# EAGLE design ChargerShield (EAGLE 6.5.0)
Dings

## Sheet 1 of 2: User Interface
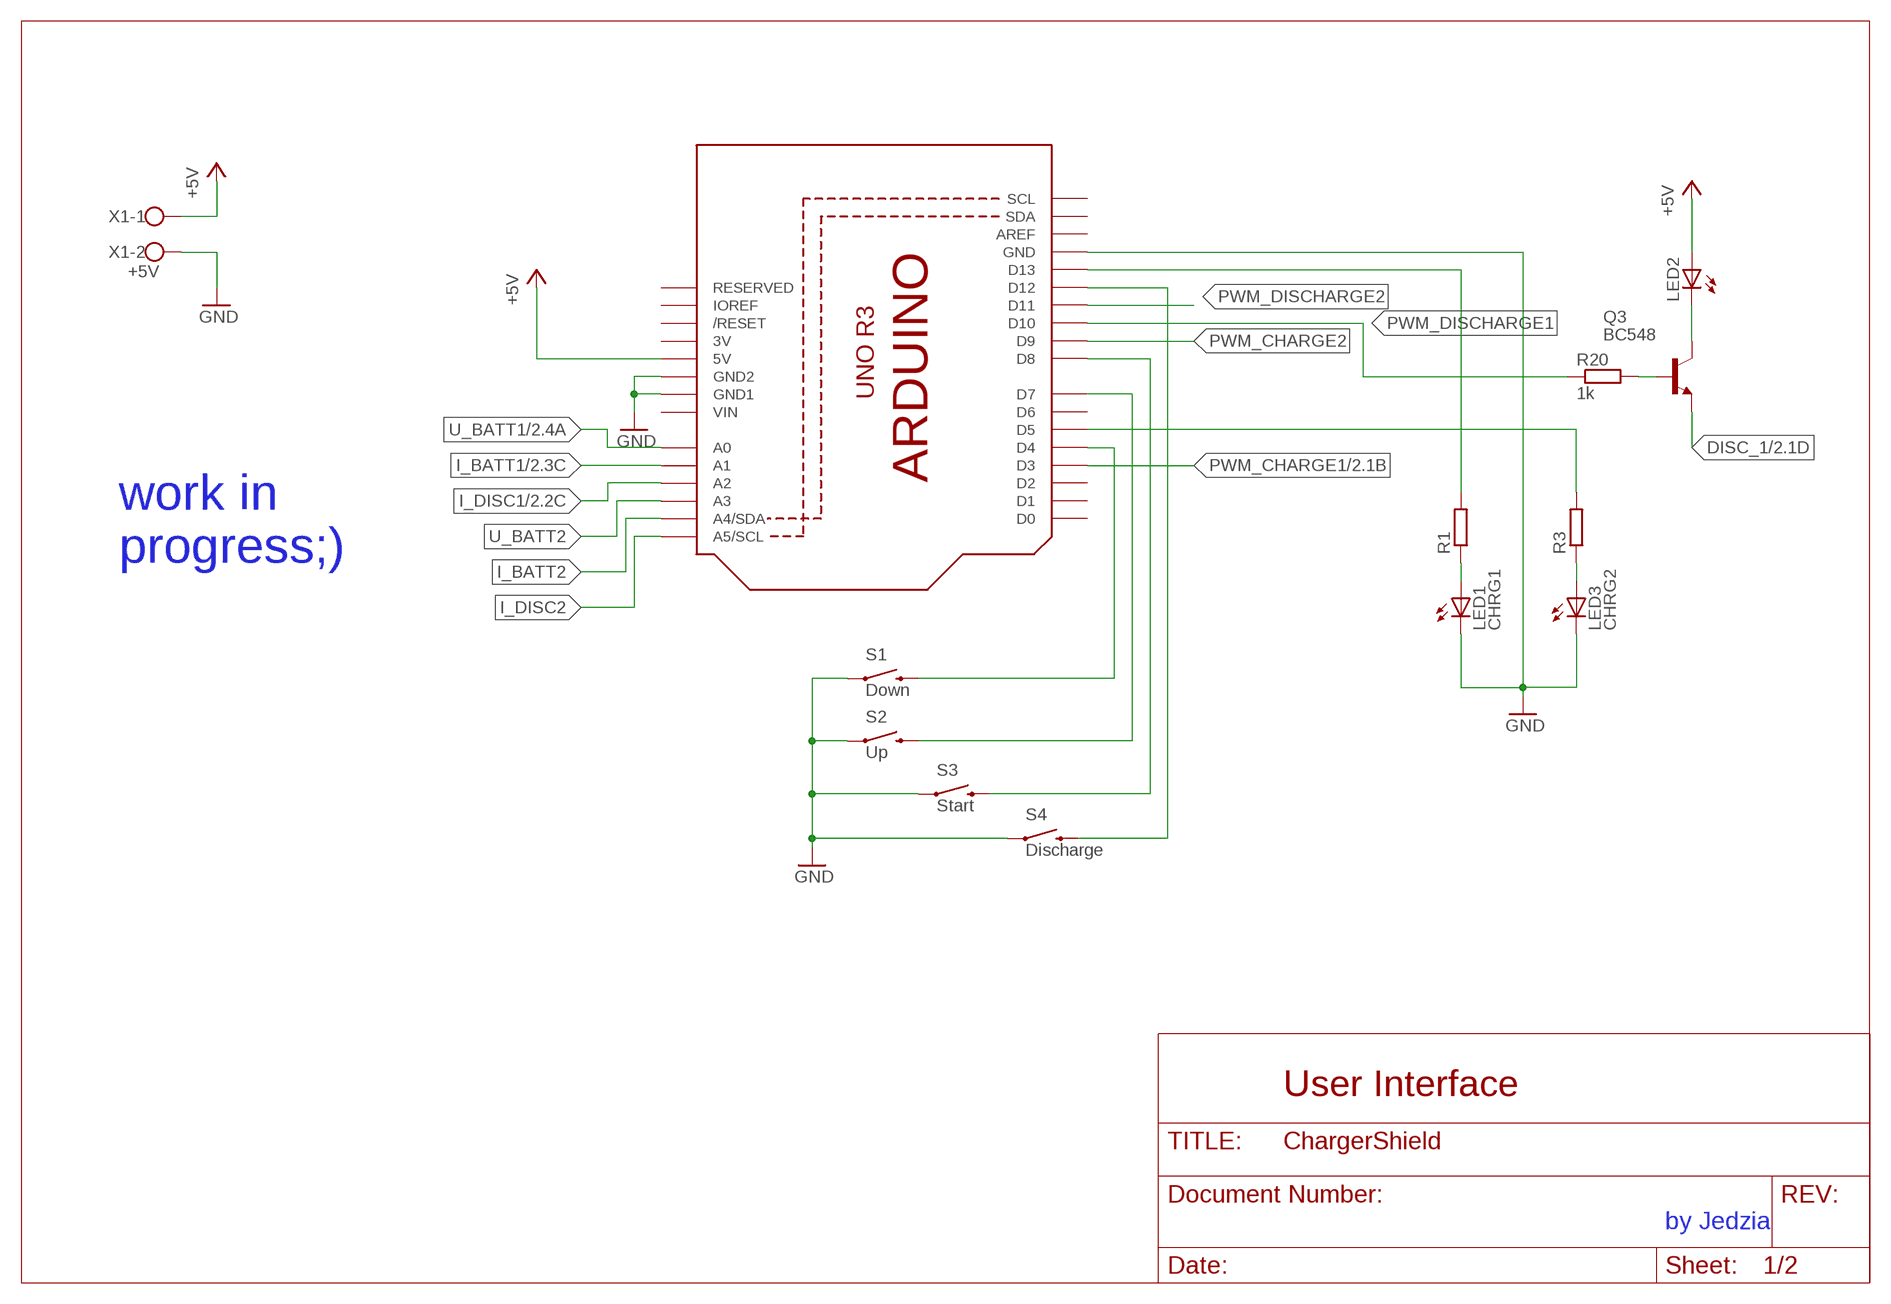
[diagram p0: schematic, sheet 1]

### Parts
LED1  CHRG1  LED5MM_BIG  [LED5MM_BIG]
LED2  LED5MM_BIG  [LED5MM_BIG]
LED3  CHRG2  LED5MM_BIG  [LED5MM_BIG]
Q3  BC548  [TO92-EBC]
R1  R-EU_0207/10  [0207/10]
R3  R-EU_0207/10  [0207/10]
R20  1k  R-EU_0204/7  [0204/7]
S1  Down  SWITCH-MOMENTARY-2PTH  [TACTILE-PTH]
S2  Up  SWITCH-MOMENTARY-2PTH  [TACTILE-PTH]
S3  Start  SWITCH-MOMENTARY-2PTH  [TACTILE-PTH]
S4  Discharge  SWITCH-MOMENTARY-2PTH  [TACTILE-PTH]
U$1  ARDUINOR3BPLACE-LONG  [ARDUINOR3-BPLACE-LONG]
X1  +5V  W237-102  [W237-102]

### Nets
+5V: LED2.A U$1.5V X1.1
DISC_1: Q3.E ; also sheet 2
GND: LED1.K(C) LED3.K(C) S1.1 S2.1 S3.1 S4.1 U$1.GND U$1.GND1 U$1.GND2 X1.2 ; also sheet 2
I_BATT1: U$1.A1 ; also sheet 2
I_BATT2: U$1.A4(A4/SDA)
I_DISC1: U$1.A2 ; also sheet 2
I_DISC2: U$1.A5(A5/SCL)
N$1: R1.2 U$1.D13
N$2: LED1.A R1.1
N$3: S1.3 U$1.D4
N$4: S2.3 U$1.D7
N$19: R3.2 U$1.D5
N$20: Q3.B R20.2
N$21: LED2.K(C) Q3.C
N$22: S3.3 U$1.D8
N$23: S4.3 U$1.D12
N$24: LED3.A R3.1
PWM_CHARGE1: U$1.D3 ; also sheet 2
PWM_CHARGE2: U$1.D9
PWM_DISCHARGE1: R20.1 U$1.D10
PWM_DISCHARGE2: U$1.D11
U_BATT1: U$1.A0 ; also sheet 2
U_BATT2: U$1.A3
Unconnected: U$1.AREF U$1.D0 U$1.D1 U$1.D2 U$1.D6 U$1.IOREF U$1.RESERVED U$1.RESET(/RESET) U$1.SCL U$1.SDA

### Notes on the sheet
- work in
  progress;)
- User Interface
- by Jedzia

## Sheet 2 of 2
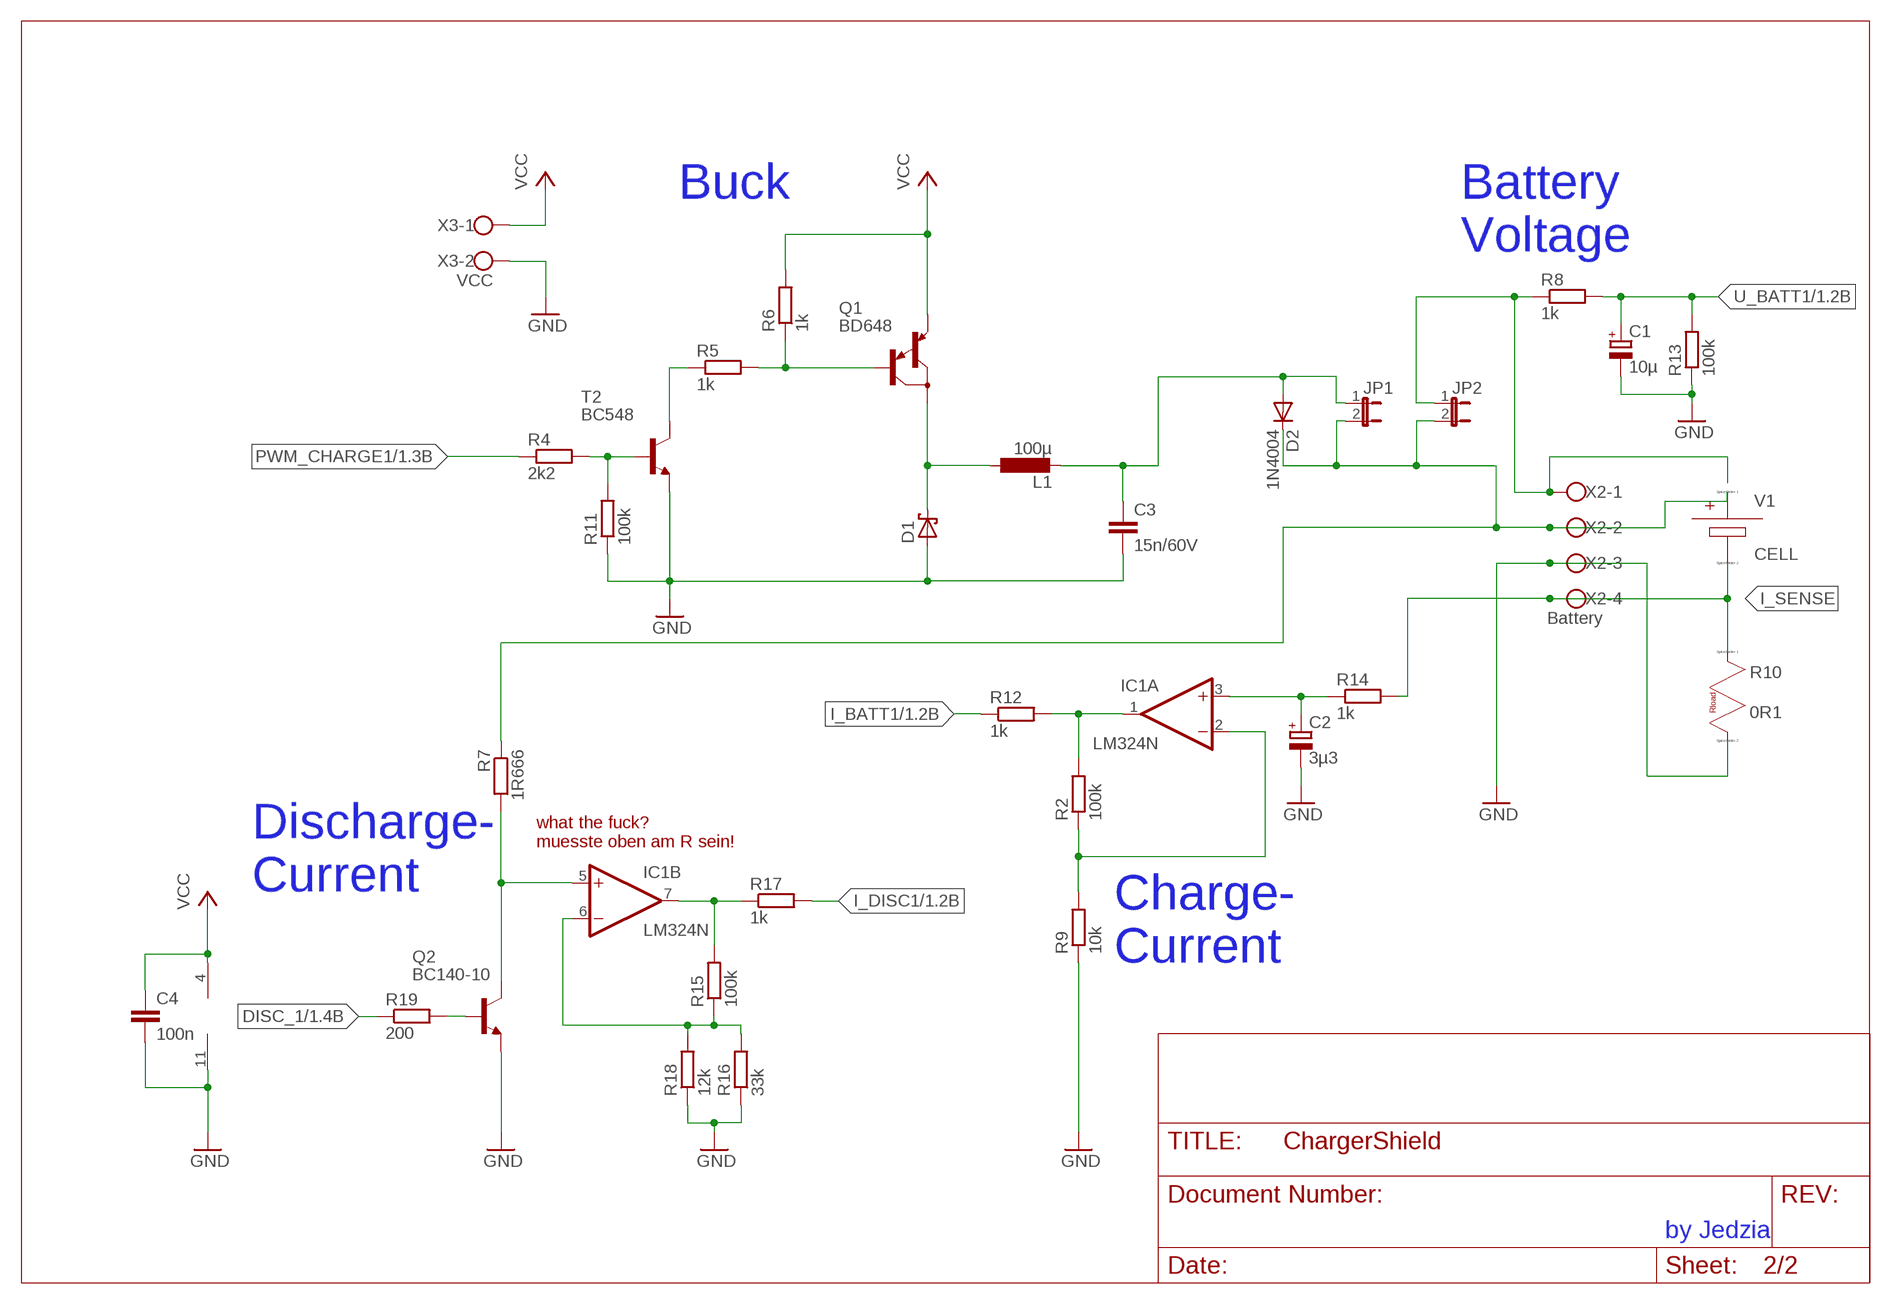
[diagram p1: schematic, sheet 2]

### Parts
C1  10µ  CPOL-EUE5-5  [E5-5]
C2  3µ3  CPOL-EUE5-5  [E5-5]
C3  15n/60V  C-EU025_050-025X075  [C025_050-025X075]
C4  100n  C-EU025_050-025X075  [C025_050-025X075]
D1  SCHOTTKY-DIODEDO35-7  [DO35-7]
D2  1N4004  [DO41-10]
IC1  LM324N  [DIL14]
JP1  JP1E  [JP1]
JP2  JP1E  [JP1]
L1  100µ  L-EU0207/12  [0207/12]
Q1  BD648  [TO220]
Q2  BC140-10  [TO39]
R2  100k  R-EU_0204/7  [0204/7]
R4  2k2  R-EU_0207/12  [0207/12]
R5  1k  R-EU_0207/15  [0207/15]
R6  1k  R-EU_0207/10  [0207/10]
R7  1R666  R-EU_0414/15  [0414/15]
R8  1k  R-EU_0207/10  [0207/10]
R9  10k  R-EU_0207/10  [0207/10]
R10  0R1  RES_RLOAD  (no package)
R11  100k  R-EU_0207/10  [0207/10]
R12  1k  R-EU_0207/10  [0207/10]
R13  100k  R-EU_0207/12  [0207/12]
R14  1k  R-EU_0207/10  [0207/10]
R15  100k  R-EU_0207/10  [0207/10]
R16  33k  R-EU_0207/10  [0207/10]
R17  1k  R-EU_0207/15  [0207/15]
R18  12k  R-EU_0207/10  [0207/10]
R19  200  R-EU_0207/10  [0207/10]
T2  BC548  BC238  [TO92]
V1  CELL  (no package)
X2  Battery  W237-4  [W237-4]
X3  VCC  W237-102  [W237-102]

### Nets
DISC_1: R19.1 ; also sheet 1
GND: C1.- C2.- C3.2 C4.2 D1.A IC1.11(P:V-) Q2.1(E) R9.1 R10.B R11.1 R13.1 R16.1 R18.1 T2.1(E) X2.3 X3.2 ; also sheet 1
I_BATT1: R12.1 ; also sheet 1
I_DISC1: R17.2 ; also sheet 1
I_SENSE: R10.A R14.2 V1.- X2.4
N$5: R4.2 R11.2 T2.2(B)
N$6: R5.1 T2.3(C)
N$7: Q1.1(B) R5.2 R6.1
N$8: JP2.1 R8.1 X2.1
N$9: D1.C L1.1 Q1.2(C)
N$10: C3.1 D2.A JP1.1 L1.2
N$11: IC1.1(A:OUT) R2.2 R12.2
N$12: IC1.5(B:+IN) Q2.3(C) R7.2
N$13: D2.C JP1.2 JP2.2 R7.1 V1.+ X2.2
N$14: IC1.2(A:-IN) R2.1 R9.2
N$15: C2.+ IC1.3(A:+IN) R14.1
N$16: IC1.6(B:-IN) R15.1 R16.2 R18.2
N$17: IC1.7(B:OUT) R15.2 R17.1
N$18: Q2.2(B) R19.2
PWM_CHARGE1: R4.1 ; also sheet 1
U_BATT1: C1.+ R8.2 R13.2 ; also sheet 1
VCC: C4.1 IC1.4(P:V+) Q1.3(E) R6.2 X3.1
Unconnected: IC1.8(C:OUT) IC1.9(C:-IN) IC1.10(C:+IN) IC1.12(D:+IN) IC1.13(D:-IN) IC1.14(D:OUT)

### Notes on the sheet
- Buck
- Battery
  Voltage
- what the fuck?
  muesste oben am R sein!
- Discharge-
  Current
- Charge-
  Current
- by Jedzia

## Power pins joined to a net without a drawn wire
3V: U$1.3V
VIN: U$1.VIN

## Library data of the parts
C1 C2 = rcl:CPOL-EU: POLARIZED CAPACITOR, European symbol
C3 C4 = rcl:C-EU: CAPACITOR, European symbol
D1 = diode:SCHOTTKY-DIODE: Schottky Diode
D2 = diode:1N4004: DIODE
IC1 = linear:LM324: OP AMP
JP1 JP2 = bigger:JP1E: JUMPER
L1 = rcl:L-EU: INDUCTOR, European symbol
LED1-LED3 = bigger:LED: LED
Q1 = transistor-pnp:BD648: PNP Darlington Transistor
Q2 = transistor-npn:BC140-10: NPN Transistor
Q3 = transistor-npn:BC548*: NPN Transistor
R1-R9 R11-R20 = rcl:R-EU_: RESISTOR, European symbol
R10 = lt-spice-simulation:RES_RLOAD: A resistor
S1-S4 = SparkFun-Electromechanical:SWITCH-MOMENTARY-2: Various NO switches- pushbuttons, reed, etc
T2 = transistor:BC238: NPN TRANSISTOR
U$1 = arduino-long:ARDUINOR3: This is a new object for the new Arduino R3 - with extra pins that you may want to use (such as IOref, and duplicated A4/A5
V1 = Misc:CELL: Voltage Source, either DC, AC, PULSE, SINE, PWL, EXP, or SFFM
X1 X3 = con-wago-500:W237-102: WAGO SCREW CLAMP; MPN: 237-102; OC_FARNELL: unknown; OC_NEWARK: 70K9898
X2 = con-wago-500:W237-4: WAGO SCREW CLAMP; OC_FARNELL: unknown; OC_NEWARK: unknown

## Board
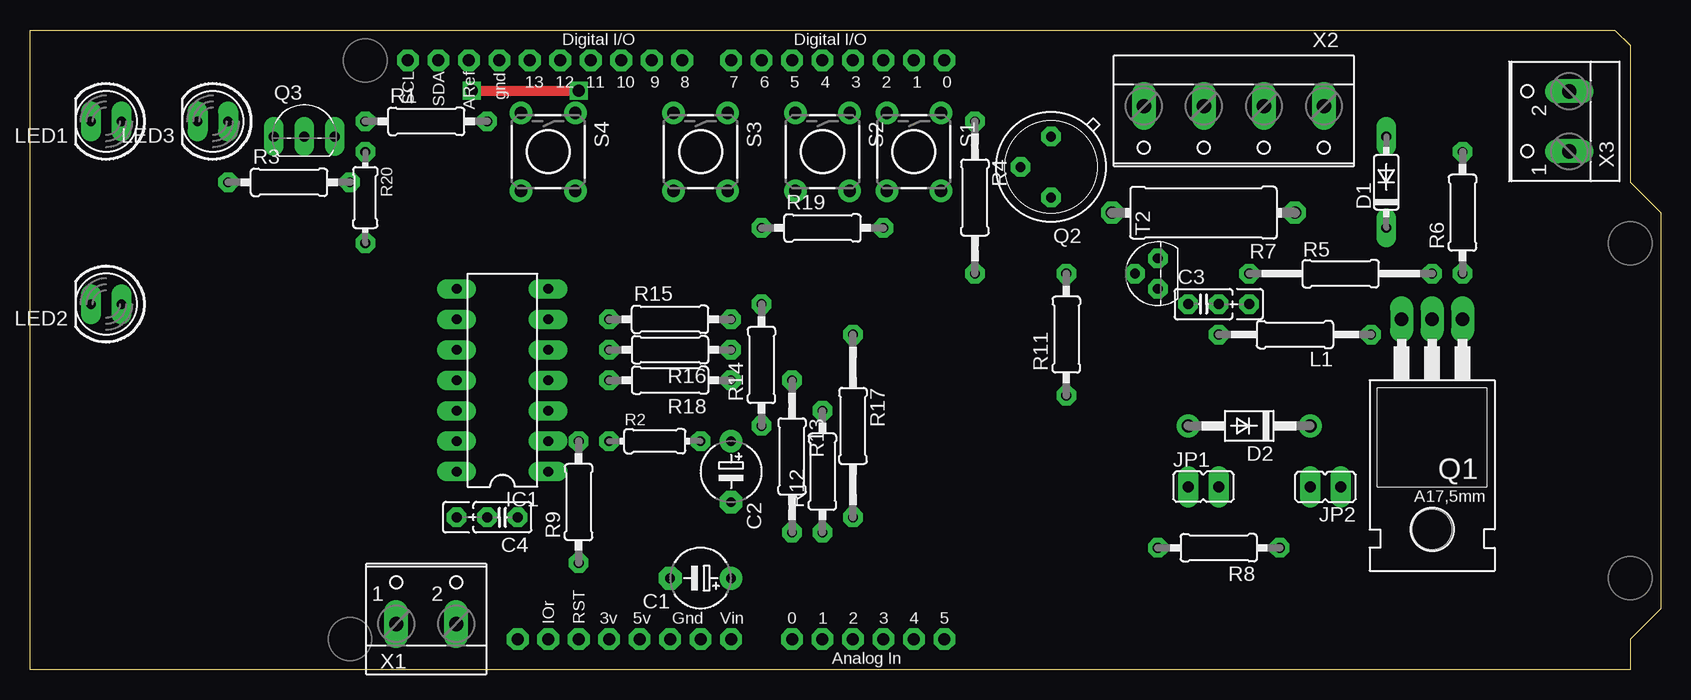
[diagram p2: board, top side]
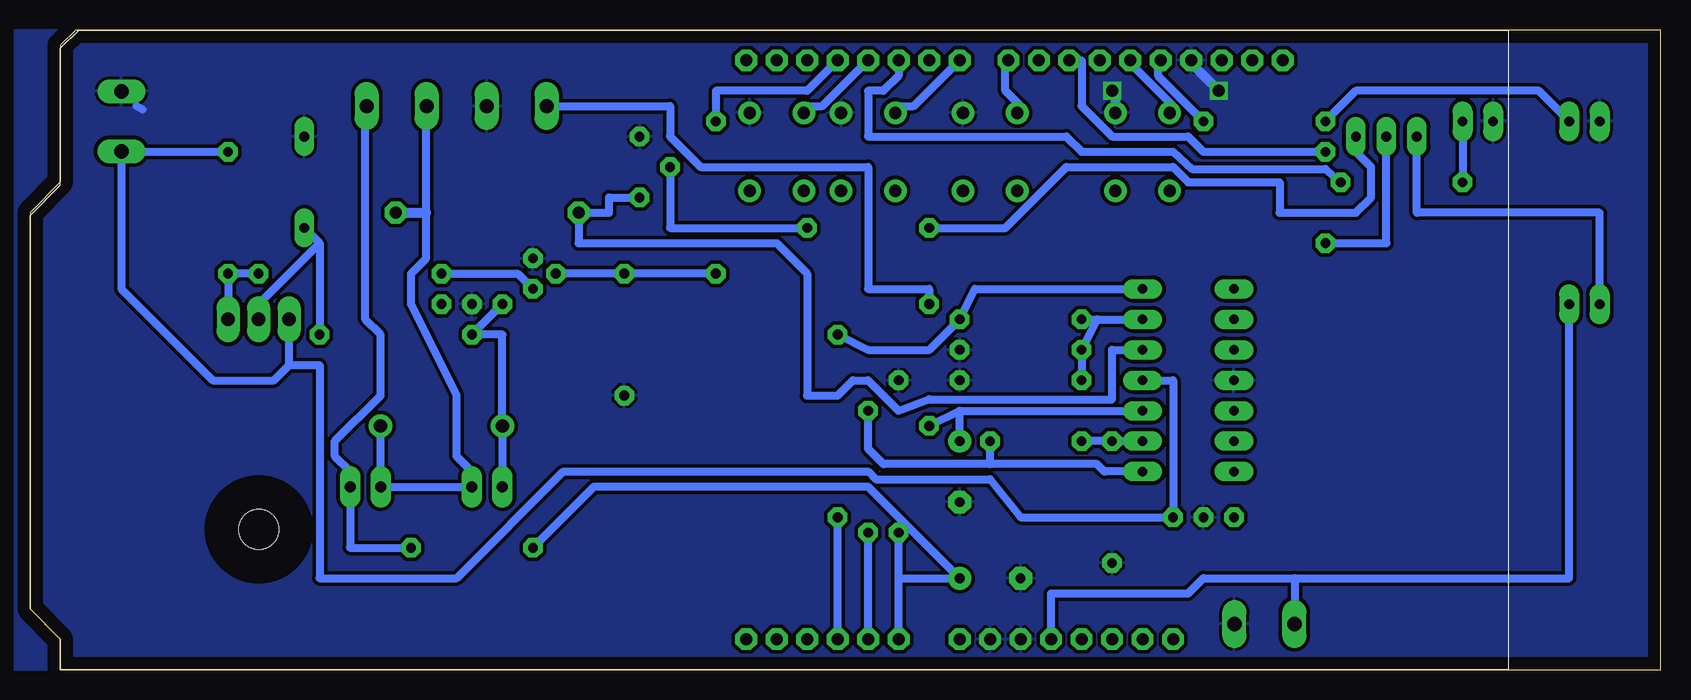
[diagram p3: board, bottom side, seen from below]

Size 135.89 x 53.34 mm. Coordinates in mm from the lower left corner, seen from the top.
Outline: 0,53.34 132.08,53.34 133.35,52.07 133.35,40.64 135.89,38.1 135.89,5.08 133.35,2.54 133.35,0 0,0 0,53.34
Copper layers (1*16): Top 0.035mm / dielectric 1.5mm / Bottom 0.035mm
Design rules "serialTTl *": minimum track width 26mil, minimum drill 24mil, track to track 8mil, track to pad 8mil, pad to pad 8mil, via to via 8mil, smd to smd 8mil, copper to edge 40mil, drill to drill 8mil, minimum pad ring 16mil, minimum via ring 8mil, stop-mask expansion 4mil, vias tented up to drill 0mil, thermal gap 10mil

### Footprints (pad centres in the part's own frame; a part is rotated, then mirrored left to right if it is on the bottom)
E5-5 = drill 0.813 pad 1.905: + -2.54,0 | drill 0.813 pad 1.905 octagon: - 2.54,0
C025_050-025X075 = drill 0.813 octagon: 1 -1.27,0; 2 1.27,0; 3 3.81,0
DO35-7 = drill 0.813 long: A 3.81,0; C -3.81,0
DO41-10 = drill 1.118: A 5.08,0; C -5.08,0
DIL14 = drill 0.813 long: 1 -7.62,-3.81; 2 -5.08,-3.81; 3 -2.54,-3.81; 4 0,-3.81; 5 2.54,-3.81; 6 5.08,-3.81; 7 7.62,-3.81; 8 7.62,3.81; 9 5.08,3.81; 10 2.54,3.81; 11 0,3.81; 12 -2.54,3.81; 13 -5.08,3.81; 14 -7.62,3.81
JP1 = drill 0.914 long: 1 0,-1.27; 2 0,1.27
0207/12 = drill 0.813 octagon: 1 -6.35,0; 2 6.35,0
LED5MM_BIG = drill 0.8 pad 1.676 long: A -1.27,0; K 1.27,0
TO220 = drill 1.118 long: 1 -2.54,-6.35; 2 0,-6.35; 3 2.54,-6.35 | hole 3.302: 0,11.176
TO39 = drill 0.813 octagon: 1 0,-2.54; 2 2.54,0; 3 0,2.54
TO92-EBC = drill 0.813 long: B 0,-1.27; C -2.54,-1.27; E 2.54,-1.27
0207/10 = drill 0.813 octagon: 1 -5.08,0; 2 5.08,0
0204/7 = drill 0.813 octagon: 1 -3.81,0; 2 3.81,0
0207/15 = drill 0.813 octagon: 1 -7.62,0; 2 7.62,0
0414/15 = drill 1.016 octagon: 1 -7.62,0; 2 7.62,0
TACTILE-PTH = drill 1.016 pad 1.88: 1 -3.251,2.261; 2 3.251,2.261; 3 -3.251,-2.261; 4 3.251,-2.261
TO92 = drill 0.813 octagon: 1 1.27,0; 2 0,1.905; 3 -1.27,0
ARDUINOR3-BPLACE-LONG = drill 1 pad 1.676 octagon: 3V 35.56,2.54; 5V 38.1,2.54; A0 50.8,2.54; A1 53.34,2.54; A2 55.88,2.54; A3 58.42,2.54; A4 60.96,2.54; A5 63.5,2.54; AREF 23.876,50.8; D0 63.5,50.8; D1 60.96,50.8; D2 58.42,50.8; D3 55.88,50.8; D4 53.34,50.8; D5 50.8,50.8; D6 48.26,50.8; D7 45.72,50.8; D8 41.656,50.8; D9 39.116,50.8; D10 36.576,50.8; D11 34.036,50.8; D12 31.496,50.8; D13 28.956,50.8; GND 26.416,50.8; GND1 43.18,2.54; GND2 40.64,2.54; IOREF 30.48,2.54; RESERVED 27.94,2.54; RESET 33.02,2.54; SCL 18.796,50.8; SDA 21.336,50.8; VIN 45.72,2.54
W237-102 = drill 1.194 long: 1 -2.5,-1.27; 2 2.5,-1.27
W237-4 = drill 1.194 long: 1 -7.5,-1.27; 2 -2.5,-1.27; 3 2.5,-1.27; 4 7.5,-1.27

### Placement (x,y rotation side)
C1  55.88,7.62 180 top
C2  58.42,16.51 270 top
C3  97.79,30.48 0 top
C4  39.37,12.7 180 top
D1  113.03,40.64 90 top
D2  101.6,20.32 180 top
IC1  39.37,24.13 90 top
JP1  97.79,15.24 270 top
JP2  107.95,15.24 90 top
L1  105.41,27.94 180 top
LED1  6.35,45.72 180 top
LED2  6.35,30.48 180 top
LED3  15.24,45.72 180 top
Q1  116.84,22.86 180 top
Q2  85.09,41.91 180 top
Q3  22.86,45.72 0 top
R1  33.02,45.72 0 top
R2  52.07,19.05 0 top
R3  21.59,40.64 0 top
R4  78.74,39.37 270 top
R5  109.22,33.02 0 top
R6  119.38,38.1 90 top
R7  97.79,38.1 180 top
R8  99.06,10.16 180 top
R9  45.72,13.97 90 top
R11  86.36,27.94 90 top
R12  66.04,16.51 90 top
R13  63.5,17.78 270 top
R14  60.96,25.4 90 top
R15  53.34,29.21 0 top
R16  53.34,26.67 180 top
R17  68.58,20.32 270 top
R18  53.34,24.13 180 top
R19  66.04,36.83 0 top
R20  27.94,39.37 270 top
S1  73.66,43.18 270 top
S2  66.04,43.18 270 top
S3  55.88,43.18 270 top
S4  43.18,43.18 270 top
T2  93.98,33.02 90 top
U$1  12.7,0 0 top
X1  33.02,5.08 0 top
X2  100.33,45.72 180 top
X3  127,45.72 90 top

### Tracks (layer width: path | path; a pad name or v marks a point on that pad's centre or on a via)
+5V
  Bottom 0.66: 30.48,7.62 38.1,7.62 39.37,6.35 50.8,6.35 U$1.5V | 30.48,7.62 7.62,7.62 LED2.A | 30.48,7.62 30.48,3.81 X1.1
DISC_1
  Bottom 0.66: Q3.E 25.4,43.18 24.13,41.91 24.13,39.37 25.4,38.1 31.75,38.1 31.75,40.64 39.37,40.64 40.64,41.91 49.53,41.91 54.61,36.83 R19.1
GND  (via drill 1)
  Top 0.813: v36.83,48.26 v45.72,48.26
  Bottom 0.66: 127,46.99 126.53,46.73
  Bottom 0.813: U$1.GND 39.37,50.8 v36.83,48.26 | v45.72,48.26 45.44,48.26 S4.1
  pour Bottom (isolate 0.305): 0,0 0,53.34 137.16,53.34 137.16,0
I_BATT1
  Bottom 0.66: U$1.A1 R12.1
I_DISC1
  Bottom 0.66: U$1.A2 R17.2
I_SENSE
  Bottom 0.66: R14.2 60.96,31.75 66.04,31.75 66.04,41.91 80.01,41.91 82.55,44.45 82.55,46.99 X2.4
N$1
  Bottom 0.66: R1.2 41.91,49.53 41.91,50.8 U$1.D13
N$2
  Bottom 0.66: R1.1 25.4,48.26 10.16,48.26 LED1.A
N$3
  Bottom 0.66: U$1.D4 69.85,46.99 71.12,46.99 S1.3
N$4
  Bottom 0.66: U$1.D7 62.23,46.99 63.5,46.99 S2.3
N$5
  Bottom 0.66: R4.2 R11.2 T2.2
N$6
  Bottom 0.66: R5.1 95.25,33.02 T2.3
N$7
  Bottom 0.66: R5.2 R6.1 Q1.1
N$8
  Bottom 0.66: R8.1 109.22,10.16 JP2.1 109.22,16.51 110.49,17.78 110.49,19.05 106.68,22.86 106.68,27.94 107.95,29.21 107.95,46.99 X2.1
N$9
  Bottom 0.66: 111.76,35.56 116.84,30.48 Q1.2 116.84,27.94 | 111.76,35.56 L1.1 | 111.76,35.56 D1.C
N$10
  Bottom 0.66: C3.1 L1.2 96.52,27.94 D2.A JP1.1
N$11
  Bottom 0.66: IC1.1 46.36,16.51 46.99,17.14 55.88,17.14 | 55.88,17.14 R2.2 | 55.88,17.14 64.77,17.14 66.04,18.41 R12.2
N$12
  Bottom 0.66: IC1.5 45.72,26.67 45.72,22.54 60.96,22.54 63.5,21.59 66.04,24.13 67.31,24.13 68.58,22.86 71.12,22.86 71.12,33.02 73.66,35.56 90.17,35.56 R7.2 87.63,38.1 87.63,39.37 Q2.3
N$13
  Bottom 0.66: D2.C JP2.2 JP1.2 99.06,16.51 100.33,17.78 100.33,22.86 104.14,30.48 104.14,33.02 102.87,34.29 102.87,38.1 102.87,44.45 X2.2
  Bottom 0.813: R7.1 102.87,38.1
N$14
  Bottom 0.66: IC1.2 R9.2 R2.1
N$15
  Bottom 0.66: 58.42,21.59 IC1.3 | C2.+ 58.42,21.59 | 58.42,21.59 R14.1
N$16
  Bottom 0.66: R18.2 R16.2 46.99,29.21 | 46.99,29.21 IC1.6 | R15.1 46.99,29.21
N$17
  Bottom 0.66: R17.1 66.04,26.67 60.96,26.67 R15.2 57.15,31.75 IC1.7
N$18
  Bottom 0.66: Q2.2 82.55,36.83 R19.2
N$19
  Bottom 0.66: U$1.D5 63.5,49.53 64.77,48.26 66.04,48.26 66.04,44.45 49.53,44.45 48.26,43.18 40.64,43.18 39.05,41.75 27.94,41.75 R3.2
N$20
  Bottom 0.66: R20.2 22.86,35.56 Q3.B
N$21
  Bottom 0.66: Q3.C 20.32,38.1 5.08,38.1 LED2.K
N$22
  Bottom 0.66: U$1.D8 54.61,50.8 54.61,48.26 53.34,46.99 S3.3
N$23
  Bottom 0.66: U$1.D12 44.45,50.8 40.64,46.99 S4.3
N$24
  Bottom 0.66: LED3.A R3.1
PWM_CHARGE1
  Bottom 0.66: U$1.D3 71.12,48.26 78.74,48.26 R4.1
PWM_DISCHARGE1
  Bottom 0.66: R20.1 38.1,43.18 39.37,44.45 45.72,44.45 48.26,46.99 48.26,50.8 U$1.D10 49.53,50.8
U_BATT1
  Bottom 0.66: U$1.A0 63.5,7.62 | 63.5,7.62 R13.2 | 63.5,7.62 C1.+ 66.04,15.24 88.9,15.24 R8.2
VCC
  Bottom 0.66: IC1.4 40.64,24.13 C4.1 53.34,12.7 55.88,15.88 65.41,15.88 66.04,16.51 91.44,16.51 100.33,7.62 111.76,7.62 111.76,25.4 114.3,25.4 | 128.27,43.18 R6.2 | 114.3,25.4 115.57,24.13 120.65,24.13 128.27,31.75 128.27,43.18 | 128.27,43.18 X3.1 | 114.3,25.4 Q1.3

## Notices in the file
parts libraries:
SparkFun-Electromechanical: Licensing: Creative Commons ShareAlike 4.0 International - https://creativecommons.org/licenses/by-sa/4.0
